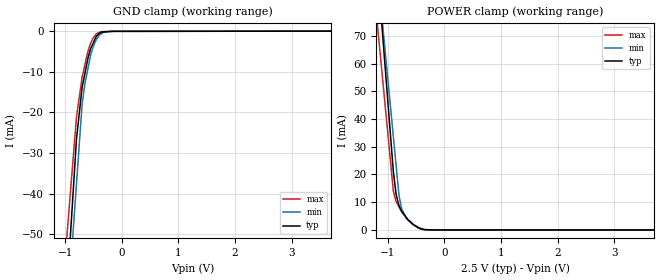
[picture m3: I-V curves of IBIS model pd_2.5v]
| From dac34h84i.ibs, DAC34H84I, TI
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[Model] pd_2.5v
Model_type Input
Vinl = 750.000mV
Vinh = 1.75000V
C_comp 1.63000pF 1.63000pF 1.63000pF
| variable typ   min   max
[Voltage Range] 2.50000V 2.25000V 2.75000V
[POWER Clamp Reference] 2.50000V 2.25000V 2.75000V
[GND Clamp Reference] 0.00000V 0.00000V 0.00000V
[Temperature Range] 25   125   -40
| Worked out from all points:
|   GND clamp passes 1 mA (typ) near -0.43 V on its own axis
|   POWER clamp passes 1 mA (typ) near -0.47 V on its own axis
[GND Clamp]
-2.5V     -404.1mA   -372.9mA   -315.9mA
-800mV    -26.55mA   -37.64mA   -21.14mA
-700mV    -13.74mA   -17.92mA   -11.26mA
-650mV    -10.26mA   -12.82mA   -8.165mA
-600mV    -6.783mA   -9.316mA   -5.075mA
-550mV    -4.26mA    -5.809mA   -2.932mA
-500mV    -2.756mA   -3.624mA   -1.515mA
-450mV    -1.251mA   -2.058mA   -667.3uA
-400mV    -546.6uA   -1.038mA   -242.9uA
-300mV    -149uA     -170.2uA   -57.59uA
-150mV    -16.19uA   -18uA      -17.76uA
5V        44.97uA    41.64uA    47.03uA
[POWER Clamp]
-2.5V     437.4mA    374.9mA    355.2mA
-1.15V    86.22mA    87.12mA    67.44mA
-1.1V     73.21mA    76.46mA    56.78mA
-1V       47.2mA     55.15mA    35.47mA
-900mV    21.19mA    33.83mA    14.15mA
-850mV    12.74mA    23.17mA    10.18mA
-800mV    8.817mA    12.52mA    8.34mA
-750mV    6.588mA    7.517mA    6.501mA
-650mV    3.907mA    3.653mA    3.836mA
-450mV    755.2uA    754.7uA    586.4uA
-300mV    104.6uA    0A         44.49uA
5V        0A         0A         0A
